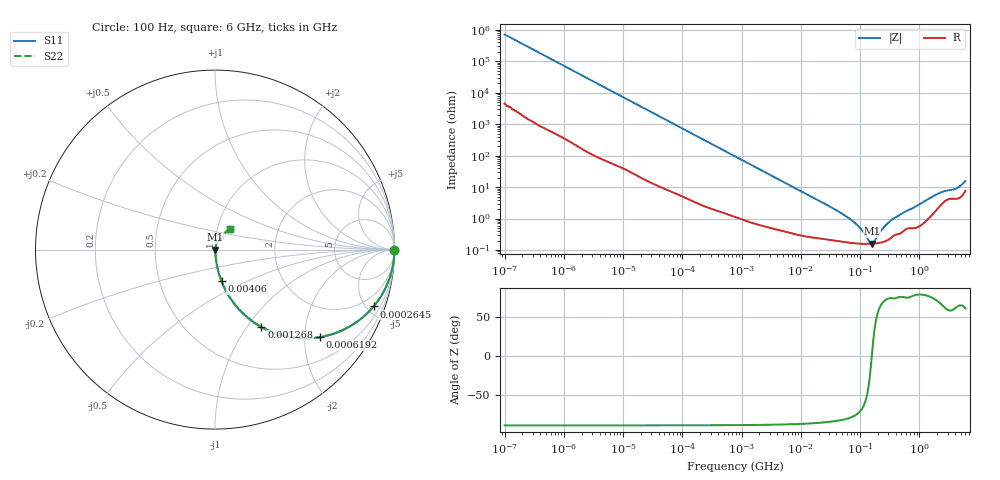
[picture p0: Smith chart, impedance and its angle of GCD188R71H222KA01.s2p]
!Murata Part Number: GCD188R71H222KA01
!These Parameters are Measured in Series Mode Connection
!Data Generated on Mar 13, 2026
!  o--ll--o
!Port1  Port2
!  o------o
!Operation Temp=25[degC], DC Bias Voltage=0[V]
!Freq. Start=100[Hz] Stop=6[GHz] 401[Steps]
# Hz S RI R 50
!Freq.(Hz) S11(Real) S11(Imag) S21(Real) S21(Imag) S12(Real) S12(Imag) S22(Real) S22(Imag)
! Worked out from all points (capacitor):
!   401 points, 100 Hz to 6 GHz, reference 50 ohm
!   read as one part in series: C = 2.22 nF near 109 Hz
!   lowest |Z| = 158 mohm at 159.6 MHz (marker M1)
!   series resonance near 158.2 MHz, so ESL is about 460 pH
!   S11 on the Smith chart (normalised r, x): 100 Hz: open; 264.5 kHz: 1.05, -5.57; 619.2 kHz: 1.03, -2.39; 1.268 MHz: 1.02, -1.17; 4.06 MHz: 1.01, -0.37; 6 GHz: 1.15, +0.27
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100  1 -0.00014  9e-07 0.00014  9e-07 0.00014  1 -0.00014
2008  1 -0.00277  2.03e-05 0.00277  2.03e-05 0.00277  1 -0.00277
40335  0.9966 -0.055  0.00336 0.055  0.00336 0.055  0.9966 -0.055
108014  0.9778 -0.1438  0.0222 0.1438  0.0222 0.1438  0.9778 -0.1438
264476  0.8837 -0.3166  0.1163 0.3166  0.1163 0.3166  0.8837 -0.3166
619225  0.5868 -0.487  0.4132 0.487  0.4132 0.487  0.5868 -0.487
774597  0.4777 -0.4937  0.5223 0.4937  0.5223 0.4937  0.4777 -0.4937
1267578  0.2585 -0.431  0.7415 0.431  0.7415 0.431  0.2585 -0.431
2169299  0.1097 -0.304  0.8903 0.304  0.8903 0.304  0.1097 -0.304
4060267  0.0369 -0.1769  0.9631 0.1769  0.9631 0.1769  0.0369 -0.1769
1.555665e7  0.00481 -0.0481  0.9952 0.0481  0.9952 0.0481  0.00481 -0.0481
7.129496e7  0.00175 -0.00877  0.9983 0.00877  0.9983 0.00877  0.00175 -0.00877
9.753859e7  0.00161 -0.00502  0.9984 0.00502  0.9984 0.00502  0.00161 -0.00502
1.459435e8  0.00156 -0.000808  0.9984 0.000808  0.9984 0.000808  0.00156 -0.000808
1.596157e8  0.00157 9.47e-05  0.9984 -9.47e-05  0.9984 -9.47e-05  0.00157 9.47e-05
1.745687e8  0.0016 0.001  0.9984 -0.001  0.9984 -0.001  0.0016 0.001
2.388273e8  0.00178 0.00432  0.9982 -0.00432  0.9982 -0.00432  0.00178 0.00432
3.124326e8  0.00226 0.00755  0.9977 -0.00755  0.9977 -0.00755  0.00226 0.00755
1.791126e9  0.0178 0.0494  0.9822 -0.0494  0.9822 -0.0494  0.0178 0.0494
2.562649e9  0.0355 0.0607  0.9645 -0.0607  0.9645 -0.0607  0.0355 0.0607
4.009986e9  0.0455 0.0692  0.9545 -0.0692  0.9545 -0.0692  0.0455 0.0692
6e9  0.0849 0.115  0.9151 -0.115  0.9151 -0.115  0.0849 0.115
